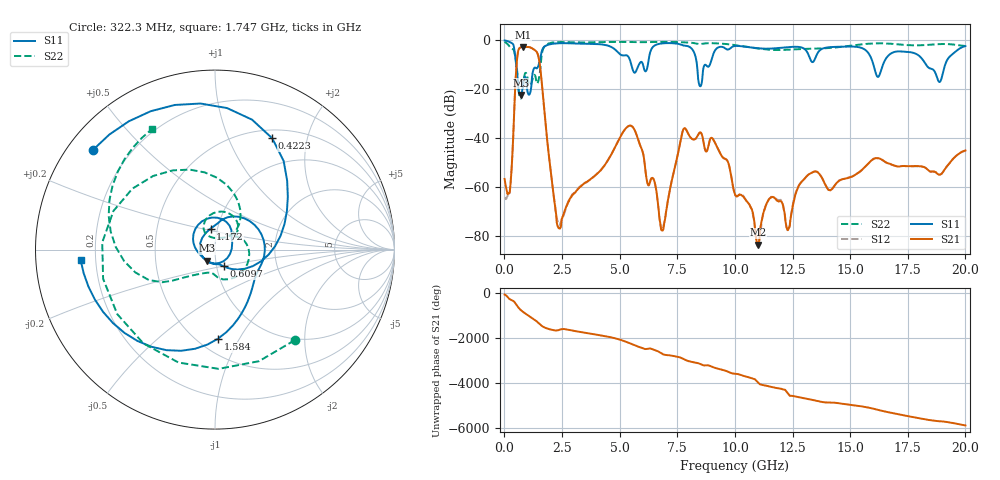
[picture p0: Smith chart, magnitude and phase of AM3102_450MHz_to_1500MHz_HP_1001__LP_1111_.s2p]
!Agilent Technologies,E8364B,MY43040894,A.07.50.67
!Agilent E8364B: A.07.50.67
!Date: Thursday, January 11, 2018 06:06:07
!Correction: S11(Full 2 Port(1,2))
!S21(Full 2 Port(1,2))
!S12(Full 2 Port(1,2))
!S22(Full 2 Port(1,2))
!S2P File: Measurements: S11, S21, S12, S22:
# Hz S  dB  R 50
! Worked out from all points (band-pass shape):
!   1601 points, 10 MHz to 20 GHz, reference 50 ohm
!   highest |S21| = -2.70 dB at 797.1 MHz (marker M1); lowest = -83.5 dB at 11 GHz (marker M2)
!   |S21| within 3 dB of the highest: 574.7 MHz to 1.45 GHz (875 MHz wide, 86.5 % of centre)
!   lowest |S11| = -22.3 dB at 709.6 MHz (marker M3), VSWR 1.17, Z = 45.3 - j5.67 ohm
!   |S11| at or under -10 dB: 516.3 MHz to 1.487 GHz (970.9 MHz wide, 96.9 % of centre); 16.01 GHz to 16.42 GHz (410.7 MHz wide, 2.53 % of centre); 18.3 GHz to 19.12 GHz (823.8 MHz wide, 4.4 % of centre)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
!   |S22| runs from -23.8 to -0.6 dB; largest |S21 - S12| = 0.0015
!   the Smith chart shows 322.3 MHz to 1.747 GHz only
!   S11 on the Smith chart (normalised r, x): 322.3 MHz: 0.07, +0.35; 422.3 MHz: 0.61, +1.46; 609.7 MHz: 1.08, -0.20; 1.172 GHz: 0.93, +0.22; 1.584 GHz: 0.62, -0.82; 1.747 GHz: 0.14, -0.04
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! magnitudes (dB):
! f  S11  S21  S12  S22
! 10 MHz  -0.1  -56.6  -64.3  -0.6
! 322.3 MHz  -1.1  -51.2  -51.2  -3.4
! 422.3 MHz  -3.1  -29.6  -29.6  -4.4
! 609.7 MHz  -19.6  -4.0  -4.0  -19.4
! 709.6 MHz  -22.3  -2.8  -2.8  -23.8
! 797.1 MHz  -18.9  -2.7  -2.7  -20.1
! 1.172 GHz  -18.5  -3.1  -3.1  -17.7
! 1.584 GHz  -6.1  -13.6  -13.6  -9.3
! 1.747 GHz  -2.5  -30.2  -30.2  -2.4
! 2.359 GHz  -1.2  -76.7  -74.9  -0.7
! 3.346 GHz  -1.4  -59.4  -59.2  -0.9
! 5.482 GHz  -9.1  -34.9  -34.9  -0.8
! 6.682 GHz  -1.5  -68.1  -68.8  -0.7
! 6.894 GHz  -1.2  -77.3  -76.2  -0.6
! 7.819 GHz  -2.2  -35.9  -35.9  -0.8
! 8.493 GHz  -18.8  -37.6  -37.6  -1.5
! 10.01 GHz  -2.3  -62.9  -63.1  -2.0
! 11 GHz  -3.2  -83.5  -83.7  -3.3
! 13.34 GHz  -8.8  -54.1  -54.0  -3.4
! 16.68 GHz  -6.1  -50.3  -50.4  -1.3
! 18.88 GHz  -17.0  -54.9  -54.8  -1.5
! 20 GHz  -2.4  -45.0  -45.1  -2.3
